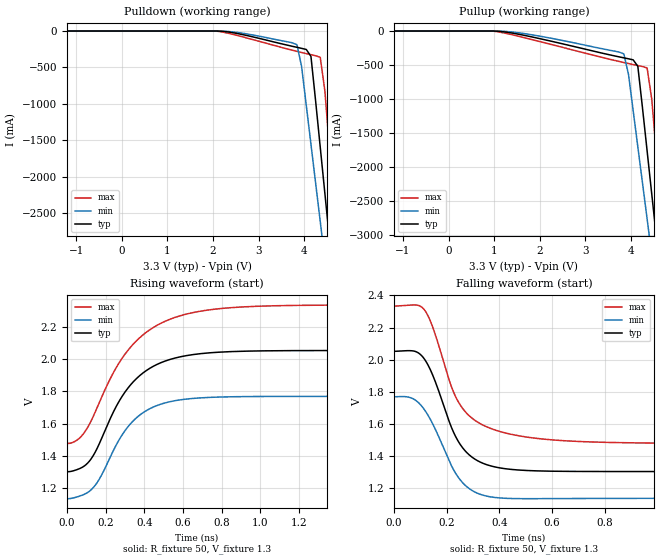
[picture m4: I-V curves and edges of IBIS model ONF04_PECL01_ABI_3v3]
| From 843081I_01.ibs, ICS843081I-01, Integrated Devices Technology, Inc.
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[Model] ONF04_PECL01_ABI_3v3
Model_type  Output_ECL
Polarity   Non-Inverting
Vmeas = 1.6
Rref = 50
Cref = 0
Vref = 1.3
|Variable  typ   min   max
C_comp   2p   1.5p   2.5p
[Voltage Range]   3.3   3.135   3.465
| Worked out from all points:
|   rising waveform, R_fixture 50, V_fixture 1.3: 20-80 % time 224ps typ, 195ps min, 270ps max; typ from 1.3 V to 2.05 V
|   falling waveform, R_fixture 50, V_fixture 1.3: 20-80 % time 112ps typ, 113ps min, 131ps max; typ from 2.05 V to 1.3 V
| Open source, no load
|  Voltage   I(typ)   I(min)   I(max)
[Pullup]
-3.3V     0A         1.541pA    0A
986.6mV   -568.5uA   -95.23uA   -3.28mA
2.007V    -113.1mA   -76.32mA   -156.3mA
3.844V    -394.3mA   -336.6mA   -463.1mA
3.946V    -408.4mA   -639.4mA   -478.1mA
4.151V    -517.8mA   -1.701A    -507.4mA
4.355V    -1.764A    -2.763A    -542.7mA
4.457V    -2.4A      -3.293A    -1.005A
4.559V    -3.036A    -3.824A    -1.816A
4.661V    -3.672A    -4.355A    -2.626A
4.763V    -4.308A    -4.886A    -3.437A
6.6V      -15.79A    -14.46A    -18.06A
[Pulldown]
-3.3V     0A         1.541pA    0A
2.109V    -725.6uA   -215.9uA   -4.017mA
3.844V    -223.7mA   -188.2mA   -278.9mA
3.946V    -237.7mA   -490.5mA   -294.3mA
4.048V    -253.1mA   -1.021A    -309.5mA
4.151V    -347.3mA   -1.551A    -324.4mA
4.355V    -1.593A    -2.612A    -360.4mA
4.457V    -2.23A     -3.142A    -823mA
4.559V    -2.866A    -3.673A    -1.634A
4.661V    -3.502A    -4.203A    -2.445A
4.763V    -4.139A    -4.734A    -3.256A
6.6V      -15.69A    -14.35A    -17.99A
[Ramp]
|   typ   min   max
dV/dt_r   0.599/0.364n   0.506/0.319n   0.685/0.439n
dV/dt_f   0.602/0.184n   0.509/0.177n   0.691/0.245n
R_load =   50.0000
[Rising Waveform]
R_fixture = 50
V_fixture = 1.3   | VCC_typ - 2V
V_fixture_max = 1.465   | VCC_max - 2V
V_fixture_min = 1.135   | VCC_min - 2V
C_fixture = 0.0p
| Time   typ   min   max
0s        1.303V     1.136V     1.477V
63ps      1.321V     1.151V     1.509V
121.8ps   1.378V     1.188V     1.61V
170.1ps   1.484V     1.263V     1.74V
235.2ps   1.661V     1.423V     1.905V
325.5ps   1.835V     1.595V     2.068V
422.1ps   1.937V     1.688V     2.175V
548.1ps   2.002V     1.739V     2.252V
936.6ps   2.048V     1.767V     2.323V
1.999ns   2.052V     1.768V     2.333V
[Falling Waveform]
R_fixture = 50
V_fixture = 1.3   | VCC_typ - 2V
V_fixture_max = 1.465   | VCC_max - 2V
V_fixture_min = 1.135   | VCC_min - 2V
C_fixture = 0.0p
| Time   typ   min   max
0s        2.052V     1.768V     2.334V
67.2ps    2.056V     1.76V      2.341V
113.4ps   2.009V     1.694V     2.315V
144.9ps   1.913V     1.607V     2.214V
216.3ps   1.587V     1.346V     1.841V
252ps     1.471V     1.25V      1.717V
317.1ps   1.371V     1.168V     1.611V
417.9ps   1.321V     1.136V     1.545V
781.2ps   1.303V     1.135V     1.486V
1.999ns   1.303V     1.136V     1.477V
